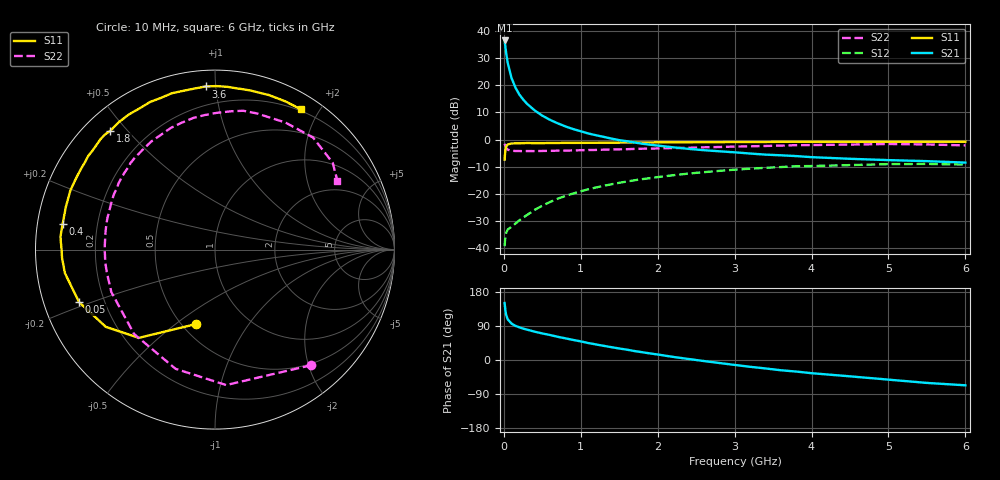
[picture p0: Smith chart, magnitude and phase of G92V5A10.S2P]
! SIEMENS Small Signal Semiconductors
! BFG235
! Si NPN RF Bipolar Junction Transistor in SOT223
! VCE = 2.5 V  IC = 100 mA
! Common Emitter S-Parameters:  July  1994
# GHz  S  MA  R  50
!  f  S11  S21  S12  S22
! GHz  MAG  ANG  MAG  ANG  MAG  ANG  MAG  ANG
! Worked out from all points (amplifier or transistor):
!   40 points, 10 MHz to 6 GHz, reference 50 ohm
!   highest |S21| = 36.5 dB at 10 MHz (marker M1)
!   |S21| within 3 dB of that: start of sweep to 23.02 MHz
!   unconditionally stable (mu >= 1): 462.4 MHz to 1.537 GHz
!   at 200 MHz: K = 0.79, MSG = 23.2 dB, |S12| = -29.8 dB
!   at 1.5 GHz: K = 1.01, MAG = 7.4 dB, |S12| = -15.9 dB
!   at 6 GHz: K = 0.92, MSG = 0.4 dB, |S12| = -9.2 dB
!   S11 on the Smith chart (normalised r, x): 10 MHz: 0.59, -0.59; 50 MHz: 0.11, -0.18; 400 MHz: 0.08, +0.08; 1.8 GHz: 0.08, +0.45; 3.6 GHz: 0.09, +0.94; 6 GHz: 0.18, +1.77
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0.01  0.4281 -104.3  66.94 150.4  0.0109 60.7  0.8381 -50.2
0.02  0.6496 -130.8  51.31 131.0  0.0165 47.1  0.7572 -85.3
0.03  0.7452 -144.7  39.44 119.4  0.0193 37.8  0.6996 -108.3
0.05  0.812 -158.9  25.94 107.4  0.022 31.4  0.6515 -133.7
0.1  0.8465 -171.1  13.61 96.0  0.0249 34.7  0.6241 -157.7
0.15  0.8535 -177.0  9.118 90.2  0.0283 40.2  0.6161 -167.5
0.2  0.8547 -180.0  6.817 86.3  0.0325 45.2  0.6157 -173.1
0.25  0.86 177.1  5.494 82.9  0.0365 48.3  0.6138 -177.1
0.3  0.864 175.1  4.586 80.2  0.0408 51.6  0.6151 179.6
0.4  0.8609 170.6  3.452 74.8  0.0507 54.5  0.6148 174.7
0.5  0.8614 167.0  2.759 70.1  0.0606 55.9  0.6181 170.6
0.7  0.8665 160.5  1.994 61.2  0.0815 55.8  0.6252 163.3
0.9  0.8696 154.9  1.566 53.0  0.1014 53.1  0.6315 157.1
1.1  0.8718 148.5  1.294 44.7  0.1218 50.0  0.6427 150.9
1.4  0.8776 141.1  1.043 33.8  0.1503 44.1  0.6572 142.4
1.8  0.8822 131.3  0.839 20.5  0.187 35.5  0.679 131.3
2.2  0.8928 122.5  0.721 8.2  0.2204 26.6  0.6991 120.5
3.2  0.9021 101.2  0.554 -17.9  0.2911 3.4  0.7518 94.4
3.6  0.9105 93.2  0.514 -27.0  0.3122 -6.5  0.7758 83.4
4.5  0.9082 77.5  0.443 -43.1  0.339 -26.0  0.8094 61.0
5.5  0.9143 64.6  0.401 -60.5  0.3564 -47.5  0.8149 36.4
6  0.9163 58.6  0.377 -66.8  0.3466 -55.7  0.7821 29.3
